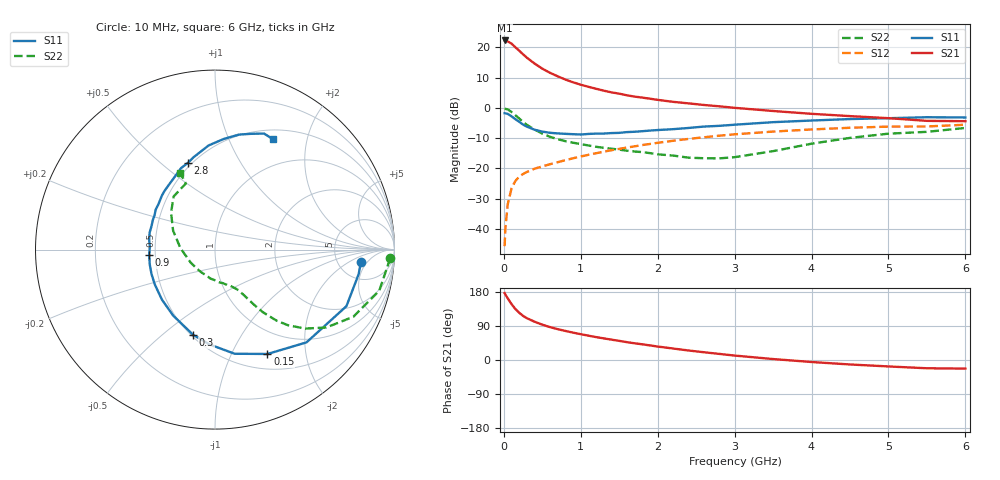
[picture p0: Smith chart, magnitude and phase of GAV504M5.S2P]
! Infineon Technologies  Discrete & RF Semiconductors
! BF775
! Si NPN RF Bipolar Junction Transistor in SOT23
! VCE = 0.5 V  IC = 4.5 mA
! Common Emitter S-Parameters:  May  1996
# GHz  S  MA  R  50
!  f  S11  S21  S12  S22
! GHz  MAG  ANG  MAG  ANG  MAG  ANG  MAG  ANG
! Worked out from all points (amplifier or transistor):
!   36 points, 10 MHz to 6 GHz, reference 50 ohm
!   highest |S21| = 22.3 dB at 10 MHz (marker M1)
!   |S21| within 3 dB of that: start of sweep to 183.1 MHz
!   unconditionally stable (mu >= 1): 670.7 MHz to end of sweep
!   at 250 MHz: K = 0.51, MSG = 19.8 dB, |S12| = -21.8 dB
!   at 1.4 GHz: K = 1.23, MAG = 6.7 dB, |S12| = -14.0 dB
!   at 6 GHz: K = 1.09, MAG = -1.2 dB, |S12| = -5.6 dB
!   S11 on the Smith chart (normalised r, x): 10 MHz: 8.45, -3.46; 150 MHz: 0.69, -1.39; 300 MHz: 0.51, -0.64; 900 MHz: 0.46, -0.03; 2.8 GHz: 0.48, +0.62; 6 GHz: 0.62, +1.47
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0.01  0.8163 -4.8  13.01 176.7  0.0052 87.2  0.9778 -2.8
0.02  0.812 -9.7  12.88 172.8  0.0102 85.5  0.965 -5.7
0.05  0.7972 -23.3  12.55 162.9  0.0255 77.2  0.9437 -14.0
0.1  0.726 -45.4  11.54 147.5  0.0469 67.3  0.8567 -25.9
0.15  0.6509 -63.3  10.04 134.5  0.0621 58.8  0.7568 -35.0
0.2  0.5906 -79.3  8.815 124.6  0.0734 53.9  0.668 -41.2
0.25  0.5296 -93.2  7.682 116.4  0.0809 50.1  0.586 -46.0
0.3  0.4907 -104.3  6.743 110.3  0.0875 48.4  0.5235 -49.1
0.4  0.4355 -122.3  5.398 101.0  0.099 46.4  0.4389 -52.6
0.5  0.4063 -136.7  4.45 93.2  0.1081 46.0  0.376 -54.7
0.6  0.3878 -149.6  3.804 86.8  0.1173 46.4  0.3331 -56.2
0.7  0.3793 -158.7  3.328 81.4  0.1267 46.9  0.3043 -57.4
0.9  0.368 -175.3  2.647 72.2  0.1474 47.4  0.2662 -59.6
1.1  0.3716 171.0  2.231 64.2  0.168 47.6  0.2399 -63.1
1.3  0.3771 159.8  1.925 57.0  0.1893 47.2  0.2191 -67.1
1.6  0.3985 146.0  1.615 47.1  0.2215 45.7  0.1964 -75.2
2.2  0.4454 124.6  1.26 30.3  0.2866 40.4  0.1632 -99.0
2.8  0.5056 107.5  1.063 16.1  0.3475 33.4  0.1467 -137.8
3.5  0.5814 93.5  0.889 2.5  0.4064 24.0  0.1931 177.4
4.5  0.6547 78.2  0.732 -11.8  0.4699 10.9  0.3197 140.0
5.5  0.7019 67.1  0.611 -21.8  0.4937 -1.9  0.4024 113.8
6  0.6947 62.2  0.603 -22.7  0.5275 -5.5  0.4669 114.4
